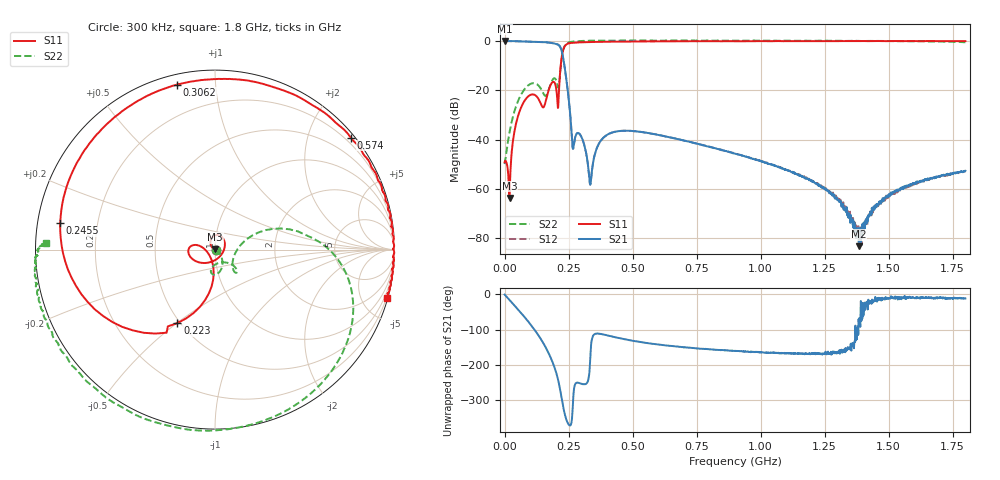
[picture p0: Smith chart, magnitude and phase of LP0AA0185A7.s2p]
!Agilent Technologies,E8358A,US40260310,A.06.04.32
!Agilent E8358A: A.06.04.32
!Date: Friday, October 18, 2019 02:03:17
!Correction: S11(Full 2 Port(1,2)) S21(Full 2 Port(1,2)) S12(Full 2 Port(1,2)) S22(Full 2 Port(1,2))
!S2P File: Measurements: S11, S21, S12, S22:
# Hz S  dB  R 50
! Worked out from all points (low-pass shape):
!   1601 points, 300 kHz to 1.8 GHz, reference 50 ohm
!   highest |S21| = 0.04 dB at 300 kHz (marker M1); lowest = -83.2 dB at 1.384 GHz (marker M2)
!   |S21| within 3 dB of the highest: start of sweep to 219.9 MHz
!   lowest |S11| = -63.6 dB at 19.42 MHz (marker M3), VSWR 1.00, Z = 50 + j0.0647 ohm
!   |S11| at or under -10 dB: start of sweep to 219.3 MHz
!   |S22| runs from -49.9 to 0.2 dB; largest |S21 - S12| = 0.0097
!   S11 on the Smith chart (normalised r, x): 300 kHz: 1.01, +0.00; 223 MHz: 0.48, -0.50; 245.5 MHz: 0.07, +0.08; 306.2 MHz: 0.05, +0.79; 574 MHz: 0.09, +2.78; 1.8 GHz: 0.09, -7.27
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300000  -49.16 4.1  0.04 -0.3  -0.05 -0.2  -49.88 2.6
1.942181e7  -63.65 99.9  -0.02 -15.7  -0.07 -15.6  -37.05 -29.0
4.079325e7  -35.45 146.0  -0.06 -32.8  -0.11 -32.8  -27.78 -43.6
6.891356e7  -25.97 120.7  -0.14 -56.1  -0.17 -56.1  -20.95 -62.2
1.251542e8  -22.43 51.5  -0.32 -108.0  -0.35 -108.0  -17.43 -97.9
1.510249e8  -26.91 -37.4  -0.42 -137.3  -0.45 -137.2  -21.10 -93.6
1.723963e8  -19.92 -132.5  -0.61 -166.6  -0.64 -166.6  -19.76 -46.1
2.072655e8  -25.62 -177.0  -1.37 124.0  -1.40 124.0  -18.00 -39.4
2.230129e8  -6.75 -117.1  -3.95 66.0  -3.97 65.9  -7.32 15.2
2.455091e8  -1.16 170.3  -18.87 -2.0  -18.90 -2.1  -0.84 -37.3
2.680054e8  -0.73 134.4  -43.66 62.6  -43.74 62.4  -0.22 -63.0
3.006249e8  -0.53 106.6  -38.94 106.9  -38.96 107.0  0.01 -83.9
3.06249e8  -0.51 103.0  -40.37 106.1  -40.40 106.1  0.03 -86.6
3.354941e8  -0.44 88.4  -58.13 -171.6  -57.78 -169.3  0.12 -98.4
3.984836e8  -0.32 68.0  -38.19 -115.4  -38.18 -115.2  0.18 -115.5
5.739544e8  -0.17 39.6  -37.52 -139.4  -37.52 -139.2  0.21 -140.4
6.009499e8  -0.14 37.0  -38.09 -141.5  -38.07 -141.8  0.19 -143.1
9.0015e8  -0.10 16.2  -45.65 -159.7  -45.59 -159.1  0.19 -160.9
1.200475e9  -0.02 3.6  -56.68 -168.4  -56.48 -168.7  0.07 -171.0
1.383819e9  -0.03 -2.7  -83.15 -77.4  -79.79 -93.7  0.03 -175.4
1.5008e9  -0.05 -6.5  -62.42 -10.6  -62.84 -13.9  0.01 -177.6
1.8e9  -0.03 -15.7  -52.58 -11.4  -52.80 -11.6  -0.53 177.9
